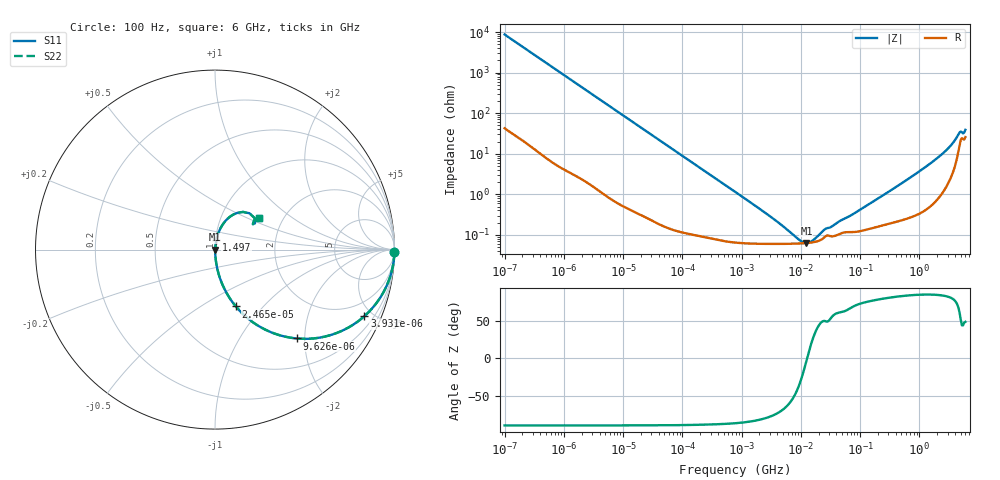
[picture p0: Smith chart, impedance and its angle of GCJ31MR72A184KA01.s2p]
!Murata Part Number: GCJ31MR72A184KA01
!These Parameters are Measured in Series Mode Connection
!Data Generated on Mar 13, 2026
!  o--ll--o
!Port1  Port2
!  o------o
!Operation Temp=25[degC], DC Bias Voltage=0[V]
!Freq. Start=100[Hz] Stop=6[GHz] 401[Steps]
# Hz S RI R 50
!Freq.(Hz) S11(Real) S11(Imag) S21(Real) S21(Imag) S12(Real) S12(Imag) S22(Real) S22(Imag)
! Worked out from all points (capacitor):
!   401 points, 100 Hz to 6 GHz, reference 50 ohm
!   read as one part in series: C = 183 nF near 109 Hz
!   lowest |Z| = 63 mohm at 12.44 MHz (marker M1)
!   series resonance near 12.77 MHz, so ESL is about 850 pH
!   S11 on the Smith chart (normalised r, x): 100 Hz: open; 3.931 kHz: 1.02, -4.48; 9.626 kHz: 1.01, -1.83; 24.65 kHz: 1.01, -0.72; 1.497 GHz: 1.01, +0.11; 6 GHz: 1.51, +0.58
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100  0.9998 -0.0115  0.000188 0.0115  0.000188 0.0115  0.9998 -0.0115
600  0.995 -0.0682  0.00498 0.0682  0.00498 0.0682  0.995 -0.0682
2008  0.9492 -0.217  0.0508 0.217  0.0508 0.217  0.9492 -0.217
3931  0.8322 -0.371  0.1678 0.371  0.1678 0.371  0.8322 -0.371
6433  0.6514 -0.4738  0.3486 0.4738  0.3486 0.4738  0.6514 -0.4738
9626  0.4566 -0.4953  0.5434 0.4953  0.5434 0.4953  0.4566 -0.4953
15752  0.2407 -0.4242  0.7593 0.4242  0.7593 0.4242  0.2407 -0.4242
24648  0.116 -0.3165  0.884 0.3165  0.884 0.3165  0.116 -0.3165
40335  0.0477 -0.2089  0.9523 0.2089  0.9523 0.2089  0.0477 -0.2089
129199  0.00576 -0.0684  0.9942 0.0684  0.9942 0.0684  0.00576 -0.0684
774597  0.00078 -0.0115  0.9992 0.0115  0.9992 0.0115  0.00078 -0.0115
3549919  0.000604 -0.00234  0.9994 0.00234  0.9994 0.00234  0.000604 -0.00234
9506416  0.000614 -0.000424  0.9994 0.000424  0.9994 0.000424  0.000614 -0.000424
1.243624e7  0.000629 -3.78e-05  0.9994 3.78e-05  0.9994 3.78e-05  0.000629 -3.78e-05
1.555665e7  0.000653 0.000284  0.9993 -0.000284  0.9993 -0.000284  0.000653 0.000284
2.545746e7  0.00089 0.00105  0.9991 -0.00105  0.9991 -0.00105  0.00089 0.00105
7.455971e7  0.00118 0.00296  0.9988 -0.00296  0.9988 -0.00296  0.00118 0.00296
3.124326e8  0.00202 0.0117  0.998 -0.0117  0.998 -0.0117  0.00202 0.0117
1.497423e9  0.00792 0.0552  0.9921 -0.0552  0.9921 -0.0552  0.00792 0.0552
3.352442e9  0.0453 0.1433  0.9547 -0.1433  0.9547 -0.1433  0.0453 0.1433
4.586474e9  0.1568 0.21  0.8432 -0.21  0.8432 -0.21  0.1568 0.21
6e9  0.2453 0.1752  0.7547 -0.1752  0.7547 -0.1752  0.2453 0.1752
